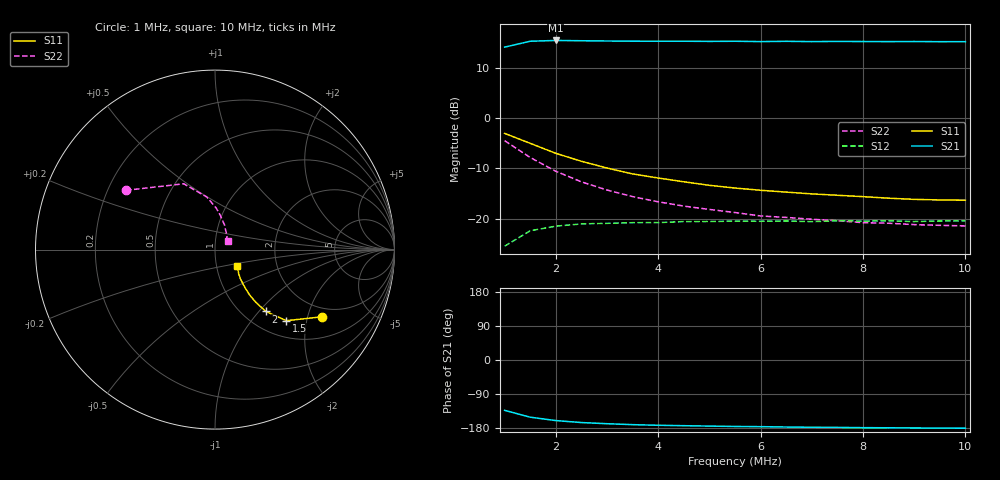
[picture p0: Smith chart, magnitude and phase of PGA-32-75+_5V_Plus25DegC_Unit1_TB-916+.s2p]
!Mini-Circuits Laboratory
!S-Parameters
!Model: PGA-32-75+
!Run / Lot / Date Code: N/A / CP621-001-03-01EV / N/A
!Fixture:
!Network Analyzer: PNA-X N5244A - 423 4 ports;  Serial number: 74314
!Date: 7/24/2017 at 7:48:00 AM
!S/N: Unit# 1
!Tested with:
# Hz  S  dB  R  50
!Frequency  S11 dB  S11 Deg  S21 dB  S21 Deg  S12 dB  S12 Deg  S22 dB  S22 Deg
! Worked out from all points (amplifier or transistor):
!   19 points, 1 MHz to 10 MHz, reference 50 ohm
!   highest |S21| = 15.5 dB at 2 MHz (marker M1)
!   |S21| within 3 dB of that: start of sweep to end of sweep
!   unconditionally stable (mu >= 1): start of sweep to end of sweep
!   at 2.5 MHz: K = 1.13, MAG = 16.1 dB, |S12| = -21.1 dB
!   at 5.5 MHz: K = 1.16, MAG = 15.5 dB, |S12| = -20.5 dB
!   at 10 MHz: K = 1.17, MAG = 15.3 dB, |S12| = -20.4 dB
!   S11 on the Smith chart (normalised r, x): 1 MHz: 1.66, -2.48; 1.5 MHz: 1.32, -1.52; 2 MHz: 1.27, -1.09; 10 MHz: 1.25, -0.23
1000000  -3.04 -32.1  14.13 -132.8  -25.48 85.6  -4.49 146.4
1500000  -5.02 -44.9  15.30 -150.9  -22.42 59.5  -7.83 115.4
2000000  -7.01 -50.6  15.46 -159.9  -21.50 44.8  -10.57 98.7
2500000  -8.59 -52.2  15.40 -165.1  -21.05 36.0  -12.68 88.4
3000000  -9.93 -52.7  15.35 -168.1  -20.94 29.7  -14.31 81.0
3500000  -11.11 -52.0  15.31 -170.6  -20.81 25.0  -15.62 74.9
4000000  -11.92 -51.1  15.30 -172.3  -20.79 22.2  -16.65 68.8
4500000  -12.67 -50.0  15.30 -173.4  -20.59 19.4  -17.51 65.0
5000000  -13.37 -49.0  15.27 -174.4  -20.57 16.5  -18.17 61.3
5500000  -13.92 -47.2  15.30 -175.4  -20.50 15.2  -18.79 56.9
6000000  -14.36 -46.1  15.23 -175.9  -20.53 13.5  -19.47 53.6
6500000  -14.73 -44.4  15.28 -176.9  -20.47 12.5  -19.76 51.6
7000000  -15.08 -42.8  15.23 -177.6  -20.61 10.4  -20.13 47.7
7500000  -15.35 -41.9  15.26 -177.9  -20.42 10.0  -20.42 45.8
8000000  -15.63 -41.0  15.24 -178.5  -20.50 9.4  -20.81 44.2
8500000  -15.93 -39.8  15.23 -178.9  -20.43 7.8  -20.92 41.8
9000000  -16.17 -38.7  15.24 -179.3  -20.58 7.5  -21.20 39.8
9500000  -16.29 -37.7  15.21 -179.7  -20.47 6.5  -21.34 37.0
1e7  -16.34 -36.7  15.22 -180.0  -20.44 6.3  -21.45 34.4
